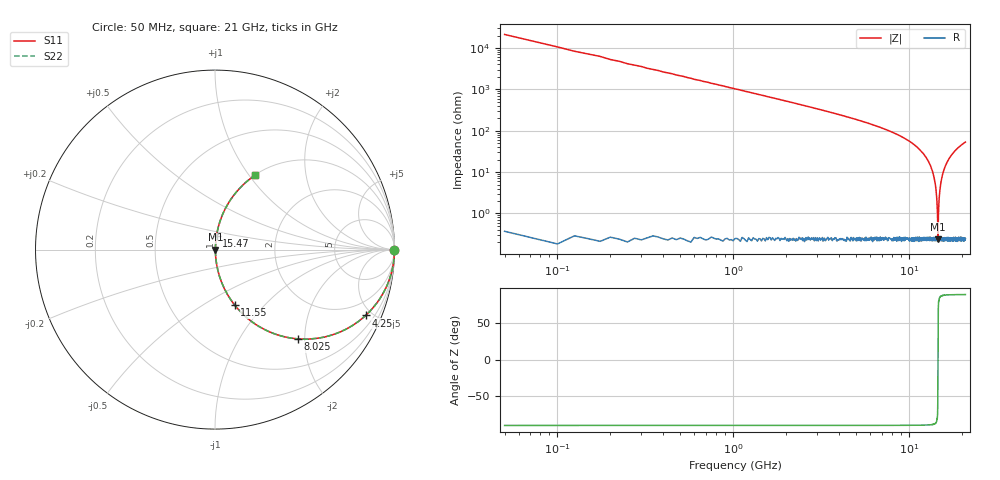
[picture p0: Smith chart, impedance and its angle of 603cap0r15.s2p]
! AVX Thin Film Operation		Date: November 2004
! Description: Accu-P® Series, Thin Film, SMD, RF Capacitor
! Part Number: 06035JR15ABT
! 50 MHz  -  10.05 GHz
! Serial Measurements
# MHZ S MA R 50
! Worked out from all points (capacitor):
!   839 points, 50 MHz to 21 GHz, reference 50 ohm
!   read as one part in series: C = 149 fF near 150 MHz
!   lowest |Z| = 238 mohm at 14.65 GHz (marker M1)
!   series resonance near 14.66 GHz, so ESL is about 790 pH
!   S11 on the Smith chart (normalised r, x): 50 MHz: open; 4.25 GHz: 1.00, -4.57; 8.025 GHz: 1.00, -1.85; 11.55 GHz: 1.01, -0.70; 15.47 GHz: 1.00, +0.16; 21 GHz: 1.00, +1.06
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50  1 -0.3  0.004712 89.7  0.004712 89.7  1 -0.3
225  1 -1.2  0.021 88.8  0.021 88.8  1 -1.2
350  0.999 -1.9  0.033 88.1  0.033 88.1  0.999 -1.9
925  0.996 -5.0  0.087 85.0  0.087 85.0  0.996 -5.0
1975  0.982 -10.7  0.186 79.2  0.186 79.2  0.982 -10.7
3550  0.942 -19.6  0.335 70.4  0.335 70.4  0.942 -19.6
4250  0.916 -23.6  0.401 66.3  0.401 66.3  0.916 -23.6
7050  0.756 -40.8  0.653 49.1  0.653 49.1  0.756 -40.8
8025  0.679 -47.1  0.733 42.7  0.733 42.7  0.679 -47.1
10525  0.438 -63.7  0.897 26.0  0.897 26.0  0.438 -63.7
11550  0.328 -70.4  0.942 19.2  0.942 19.2  0.328 -70.4
13100  0.161 -79.9  0.985 9.2  0.985 9.2  0.161 -79.9
14025  0.064 -84.2  0.996 3.7  0.996 3.7  0.064 -84.2
14400  0.026 -83.2  0.997 1.5  0.997 1.5  0.026 -83.2
14650  0.002564 -20.5  0.998 0.1  0.998 0.1  0.002564 -20.5
14725  0.006903 69.3  0.998 -0.4  0.998 -0.4  0.006903 69.3
14850  0.019 81.6  0.997 -1.1  0.997 -1.1  0.019 81.6
14975  0.031 83.8  0.997 -1.8  0.997 -1.8  0.031 83.8
15475  0.078 83.8  0.995 -4.5  0.995 -4.5  0.078 83.8
16250  0.147 80.6  0.987 -8.5  0.987 -8.5  0.147 80.6
17525  0.251 74.9  0.966 -14.5  0.966 -14.5  0.251 74.9
21000  0.469 61.8  0.881 -27.9  0.881 -27.9  0.469 61.8
